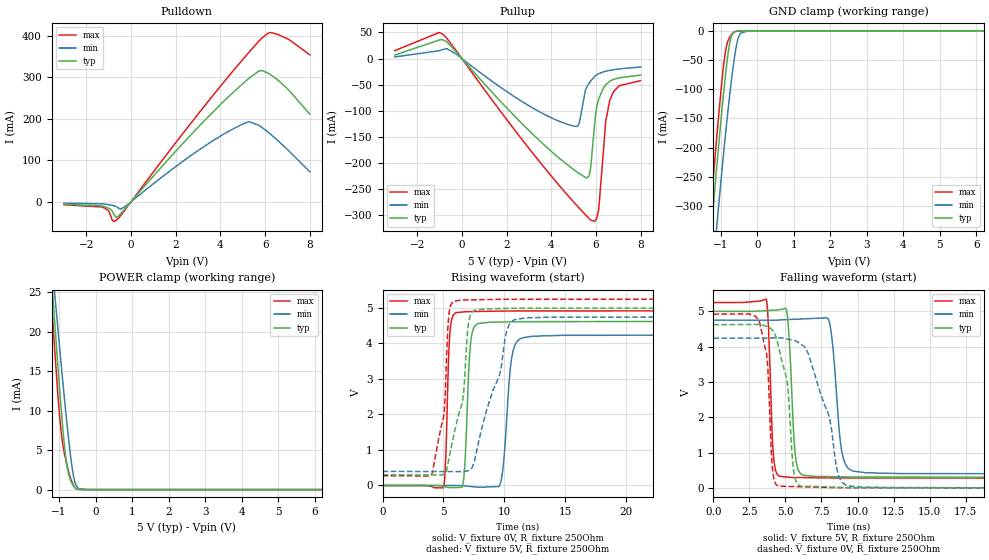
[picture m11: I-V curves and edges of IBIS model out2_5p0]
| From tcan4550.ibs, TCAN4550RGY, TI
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|   out2_5p0 Model
[Model]   out2_5p0
Model_type   3-state
Polarity   Non-Inverting
Vmeas = 2.5
Vref = 0
Cref = 2pF
Rref = 100000
|   typ   min   max
C_comp   6.445pF   6.021pF   6.601pF
|  Where Nom  PVT is Nominal Process, 5V, 27C
|   Fast PVT is Strong Process,  5.25, -40C
|   Slow PVT is Weak Process,   4.75V, 150C
[Voltage Range]   5   4.75   5.25
|Junction Temperature
[Temperature Range]   27   150   -40
[Pullup Reference]   5   4.75   5.25
[Pulldown Reference]   0   0   0
[Power Clamp Reference]   5   4.75   5.25
[GND Clamp Reference]   0   0   0
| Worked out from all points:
|   slope of the pulldown table from 0 to 0.75 V, typ, clamps not added: 16.1 ohm
|   slope of the pullup table from 0 to 0.75 V, typ, clamps not added: 20.6 ohm
|   GND clamp passes 1 mA (typ) near -0.60 V on its own axis
|   POWER clamp passes 1 mA (typ) near -0.67 V on its own axis
|   falling waveform, V_fixture 5V, R_fixture 250Ohm: 20-80 % time 334ps typ, 510ps min, 257ps max; typ from 5 V to 0.302 V
|   rising waveform, V_fixture 0V, R_fixture 250Ohm: 20-80 % time 345ps typ, 538ps min, 258ps max; typ from 0 V to 4.62 V
|   rising waveform, V_fixture 5V, R_fixture 250Ohm: 20-80 % time 1.18ns typ, 2.04ns min, 749ps max; typ from 0.302 V to 5 V
|   falling waveform, V_fixture 0V, R_fixture 250Ohm: 20-80 % time 767ps typ, 1.55ns min, 415ps max; typ from 4.62 V to 0 V
[Pulldown]
|   Voltage   I(typ)   I(min)   I(max)
-3V       -6.198mA   -3.322mA   -7.349mA
-1.317V   -10.07mA   -5.19mA    -12.58mA
-998mV    -15.71mA   -7.157mA   -22.3mA
-789mV    -28.06mA   -9.366mA   -47.19mA
-591mV    -36.18mA   -14.24mA   -41.79mA
-239mV    -14.93mA   -10.56mA   -17.27mA
4.26V     248mA      166.5mA    295.6mA
5.283V    297.9mA    193.2mA    360.8mA
5.778V    316.2mA    182.3mA    390.8mA
6.152V    309.7mA    167.1mA    406.9mA
6.581V    293.2mA    147mA      403.5mA
8V        211.3mA    72.48mA    354.4mA
[GND Clamp]
|   Voltage   I(typ)   I(min)   I(max)
-3V       -1.787A    -1.824A    -1.779A
-1.537V   -564.5mA   -655.4mA   -521.4mA
-1.262V   -347mA     -447.2mA   -298.1mA
-1.229V   -321.9mA   -422.9mA   -272.5mA
-1.097V   -225mA     -328.3mA   -174.4mA
-954mV    -128.1mA   -231.7mA   -78.72mA
-866mV    -74.34mA   -176.2mA   -33.94mA
-734mV    -15.31mA   -99.82mA   -9.032mA
-602mV    -1.078mA   -37.05mA   -1.282mA
-459mV    -34.02uA   -3.945mA   -29.01uA
-239mV    0A         -15.58uA   0A
8V        0A         0A         0A
[Pullup]
|   Voltage   I(typ)   I(min)   I(max)
-3V       6.669mA    3.027mA    15.13mA
-888mV    36.52mA    16.91mA    47.83mA
4.997V    -213.2mA   -129.9mA   -275.5mA
5.25V     -221mA     -123.9mA   -287.5mA
5.569V    -229.3mA   -56.99mA   -302.1mA
5.756V    -212.7mA   -43.63mA   -310.3mA
5.943V    -124.5mA   -34.52mA   -312.9mA
6.119V    -78.38mA   -29.29mA   -291mA
6.438V    -50.53mA   -24.41mA   -120.8mA
6.614V    -43.85mA   -22.79mA   -81.31mA
7.032V    -37.2mA    -20.08mA   -52.4mA
8V        -31.87mA   -16.24mA   -42.61mA
[POWER Clamp]
|   Voltage   I(typ)   I(min)   I(max)
-3V       155.6mA    128.7mA    164.6mA
-1.218V   27.88mA    30.1mA     24.84mA
-1.163V   24.19mA    27.21mA    20.89mA
-1.108V   20.57mA    24.34mA    17.06mA
-1.009V   14.27mA    19.27mA    10.74mA
-943mV    10.33mA    15.96mA    7.398mA
-811mV    3.932mA    9.64mA     3.677mA
-756mV    2.375mA    7.19mA     2.613mA
-668mV    1.014mA    3.702mA    1.225mA
-536mV    132.5uA    547.2uA    135.2uA
-239mV    0A         472.2nA    0A
8V        0A         0A         0A
[Ramp]
R_load = 250
|   typ   min   max
dV/dt_r   2.77328/3.42352e-10   2.54385/5.33487e-10   2.95246/2.57557e-10
dV/dt_f   2.8191/3.32918e-10   2.61217/5.07415e-10   2.98466/2.56347e-10
[Falling Waveform]
V_fixture = 5V
V_fixture_min = 4.75V
V_fixture_max = 5.25V
R_fixture = 250Ohm
C_fixture = 0F
|   Time   V(typ)   V(min)   V(max)
0s        5V         4.75V      5.25V
3.668ns   5.021V     4.749V     5.346V
4.151ns   5.032V     4.749V     995.1mV
4.589ns   5.049V     4.756V     328.6mV
5.133ns   4.888V     4.766V     305.8mV
5.67ns    984mV      4.775V     294mV
6.198ns   363.1mV    4.785V     291.5mV
8.029ns   317.7mV    4.719V     282.7mV
9.649ns   307.8mV    479.8mV    280mV
30ns      301.5mV    396.4mV    275.6mV
[Rising Waveform]
V_fixture = 0V
V_fixture_min = 0V
V_fixture_max = 0V
R_fixture = 250Ohm
C_fixture = 0F
|   Time   V(typ)   V(min)   V(max)
0s        527.7nV    8.187uV    177.5nV
5ns       -30.08mV   181uV      -66.78mV
5.522ns   -59.89mV   199.1uV    4.226V
6.015ns   -56.42mV   216.1uV    4.864V
6.64ns    101mV      -9.026mV   4.889V
7.218ns   3.95V      -27.42mV   4.9V
7.813ns   4.556V     -46.36mV   4.903V
9.636ns   4.603V     11.62mV    4.913V
11.39ns   4.615V     4.148V     4.917V
30ns      4.622V     4.24V      4.921V
[Rising Waveform]
V_fixture = 5V
V_fixture_min = 4.75V
V_fixture_max = 5.25V
R_fixture = 250Ohm
C_fixture = 0F
|   Time   V(typ)   V(min)   V(max)
0s        301.5mV    396.4mV    275.6mV
4.068ns   296.1mV    393.8mV    329mV
5.031ns   313.5mV    393.2mV    1.963V
5.424ns   693.6mV    392.9mV    4.709V
5.868ns   1.435V     392.7mV    5.192V
6.612ns   2.46V      392.2mV    5.227V
6.993ns   4.35V      413.8mV    5.229V
7.242ns   4.814V     462.8mV    5.23V
10.82ns   4.992V     4.667V     5.246V
30ns      5V         4.75V      5.25V
[Falling Waveform]
|Gnd
V_fixture = 0V
V_fixture_min = 0V
V_fixture_max = 0V
R_fixture = 250Ohm
C_fixture = 0F
|   Time   V(typ)   V(min)   V(max)
0s        4.622V     4.24V      4.921V
3.174ns   4.628V     4.244V     4.725V
3.738ns   4.572V     4.245V     3.612V
4.129ns   4.451V     4.245V     432.7mV
4.495ns   4.044V     4.246V     49.35mV
5.133ns   2.95V      4.214V     41.82mV
5.573ns   472mV      4.177V     36.97mV
6.027ns   53.39mV    4.082V     31.96mV
9.234ns   10.96mV    66.36mV    4.292mV
30ns      533.2nV    8.192uV    177.6nV
